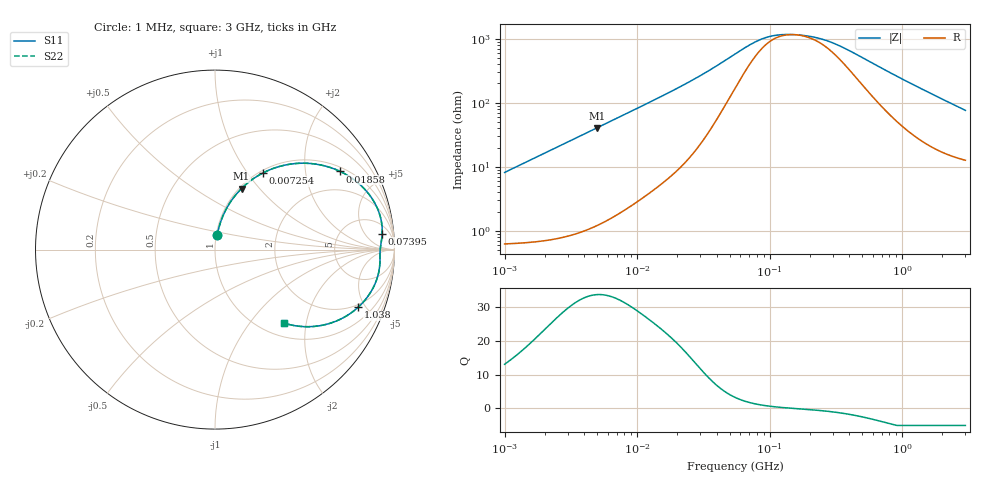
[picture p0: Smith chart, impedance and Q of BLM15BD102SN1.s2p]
! BLM15BD102SN1
# Hz S RI R 50
!Freq.(Hz) S11(Real) S11(Imag) S21(Real) S21(Imag) S12(Real) S12(Imag) S22(Real) S22(Imag)
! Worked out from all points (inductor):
!   401 points, 1 MHz to 3 GHz, reference 50 ohm
!   read as one part in series: L = 1.3 uH near 1.041 MHz
!   highest Q = 33.5 at 4.959 MHz (marker M1), where L = 1.3 uH
!   self-resonance near 153.7 MHz
!   S11 on the Smith chart (normalised r, x): 1 MHz: 1.01, +0.16; 7.254 MHz: 1.04, +1.18; 18.58 MHz: 1.15, +3.09; 73.95 MHz: 10, +14; 1.038 GHz: 1.81, -4.44; 3 GHz: 1.25, -1.50
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1000000  0.0127 0.0799  0.9873 -0.0799  0.9873 -0.0799  0.0127 0.0799
2014875  0.0327 0.1577  0.9673 -0.1577  0.9673 -0.1577  0.0327 0.1577
3823119  0.0956 0.279  0.9044 -0.279  0.9044 -0.279  0.0956 0.279
4959344  0.1478 0.3403  0.8522 -0.3403  0.8522 -0.3403  0.1478 0.3403
7254166  0.2657 0.4264  0.7343 -0.4264  0.7343 -0.4264  0.2657 0.4264
1.040059e7  0.4224 0.4766  0.5776 -0.4766  0.5776 -0.4766  0.4224 0.4766
1.461624e7  0.5881 0.4717  0.4119 -0.4717  0.4119 -0.4717  0.5881 0.4717
1.858443e7  0.6971 0.4357  0.3029 -0.4357  0.3029 -0.4357  0.6971 0.4357
2.41077e7  0.7946 0.3737  0.2054 -0.3737  0.2054 -0.3737  0.7946 0.3737
3.127247e7  0.8648 0.2992  0.1352 -0.2992  0.1352 -0.2992  0.8648 0.2992
5.477226e7  0.9287 0.1466  0.0713 -0.1466  0.0713 -0.1466  0.9287 0.1466
7.395247e7  0.9313 0.0872  0.0687 -0.0872  0.0687 -0.0872  0.9313 0.0872
9.402997e7  0.9277 0.0518  0.0723 -0.0518  0.0723 -0.0518  0.9277 0.0518
1.171891e8  0.9238 0.0263  0.0762 -0.0263  0.0762 -0.0263  0.9238 0.0263
1.550909e8  0.9204 -0.000854  0.0796 0.000854  0.0796 0.000854  0.9204 -0.000854
2.094008e8  0.9193 -0.0292  0.0807 0.0292  0.0807 0.0292  0.9193 -0.0292
3.252521e8  0.9183 -0.0812  0.0817 0.0812  0.0817 0.0812  0.9183 -0.0812
5.364635e8  0.9005 -0.168  0.0995 0.168  0.0995 0.168  0.9005 -0.168
8.005644e8  0.853 -0.2589  0.147 0.2589  0.147 0.2589  0.853 -0.2589
1.038491e9  0.7969 -0.3218  0.2031 0.3218  0.2031 0.3218  0.7969 -0.3218
1.818868e9  0.5993 -0.4212  0.4007 0.4212  0.4007 0.4212  0.5993 -0.4212
3e9  0.3853 -0.4096  0.6147 0.4096  0.6147 0.4096  0.3853 -0.4096
